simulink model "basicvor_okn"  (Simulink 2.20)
settings: Solver=ode45  StartTime=0  StopTime=10  MaxStep=.1  RelTol=1e-3  AbsTol=1e-3
undefined symbols (not defined in the file or in its folder): sfuny

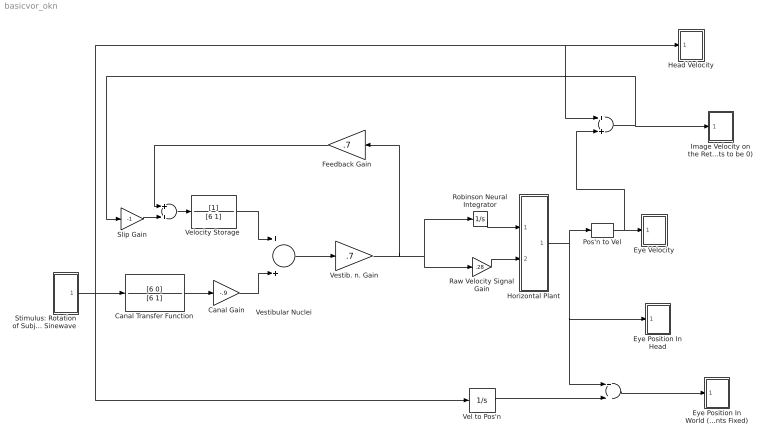
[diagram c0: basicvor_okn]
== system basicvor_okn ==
  " " : Sum  Inputs=++
  "  " : Sum  Inputs=++
  "   " : Sum  Inputs=++
  Canal Transfer Function : TransferFcn  Numerator=[6 0]  Denominator=[6 1]
  Canal Gain : Gain  Gain=-.9
  Eye Position In Head : Subsystem  LoadFcn=sfuny([],[],[],'LoadBlock')  StartFcn=sfuny([],[],[],'Start')  StopFcn=sfuny([],[],[],'Stop')  mask(Graph scope.){}
      mask help: Graph scope using MATLAB graph window. Enter plotting ranges and line type.
      mask init:
      | color = @4; ax = [0, @1, @2, @3]; dt = -1;
  Eye Position In World (Wants Fixed) : Subsystem  LoadFcn=sfuny([],[],[],'LoadBlock')  StartFcn=sfuny([],[],[],'Start')  StopFcn=sfuny([],[],[],'Stop')  mask(Graph scope.){}
      mask help: Graph scope using MATLAB graph window. Enter plotting ranges and line type.
      mask init:
      | color = @4; ax = [0, @1, @2, @3]; dt = -1;
  Eye Velocity : Subsystem  LoadFcn=sfuny([],[],[],'LoadBlock')  StartFcn=sfuny([],[],[],'Start')  StopFcn=sfuny([],[],[],'Stop')  mask(Graph scope.){}
      mask help: Graph scope using MATLAB graph window. Enter plotting ranges and line type.
      mask init:
      | color = @4; ax = [0, @1, @2, @3]; dt = -1;
  Feedback Gain : Gain  Orientation=left  Gain=.7
  Head Velocity : Subsystem  LoadFcn=sfuny([],[],[],'LoadBlock')  StartFcn=sfuny([],[],[],'Start')  StopFcn=sfuny([],[],[],'Stop')  mask(Graph scope.){}
      mask help: Graph scope using MATLAB graph window. Enter plotting ranges and line type.
      mask init:
      | color = @4; ax = [0, @1, @2, @3]; dt = -1;
  Horizontal Plant : Subsystem
  Image Velocity on the Retina (wants to be 0) : Subsystem  LoadFcn=sfuny([],[],[],'LoadBlock')  StartFcn=sfuny([],[],[],'Start')  StopFcn=sfuny([],[],[],'Stop')  mask(Graph scope.){}
      mask help: Graph scope using MATLAB graph window. Enter plotting ranges and line type.
      mask init:
      | color = @4; ax = [0, @1, @2, @3]; dt = -1;
  Pos'n to Vel : Derivative
  Raw Velocity Signal Gain : Gain  Gain=.28
  Robinson Neural Integrator : Integrator  ExternalReset=none  InitialConditionSource=internal  InitialCondition=0  LimitOutput=off  UpperSaturationLimit=inf  LowerSaturationLimit=-inf  ShowSaturationPort=off  ShowStatePort=off  AbsoluteTolerance=auto
  Slip Gain : Gain  Gain=-1
  Stimulus: Rotation of Subject Either Velocity Step or Sinewave : Subsystem
  Vel to Pos'n : Integrator  ExternalReset=none  InitialConditionSource=internal  InitialCondition=0  LimitOutput=off  UpperSaturationLimit=inf  LowerSaturationLimit=-inf  ShowSaturationPort=off  ShowStatePort=off  AbsoluteTolerance=auto
  "Velocity Storage " : TransferFcn  Numerator=[1]  Denominator=[6 1]
  Vestib. n. Gain : Gain  Gain=.7
  Vestibular Nuclei : Sum  Inputs=++
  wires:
  Canal Gain/1 -> Vestibular Nuclei/2
  Canal Transfer Function/1 -> Canal Gain/1
  "Velocity Storage "/1 -> Vestibular Nuclei/1
  Vestibular Nuclei/1 -> Vestib. n. Gain/1
  Vestib. n. Gain/1 -> Feedback Gain/1, Raw Velocity Signal Gain/1, Robinson Neural Integrator/1
  Raw Velocity Signal Gain/1 -> Horizontal Plant/2(in_2)
  Robinson Neural Integrator/1 -> Horizontal Plant/1(in_1)
  Horizontal Plant/1(out_1) -> Pos'n to Vel/1, Eye Position In Head/1(x), "   "/1
  Pos'n to Vel/1 -> Eye Velocity/1(x), "  "/2
  Stimulus: Rotation of Subject Either Velocity Step or Sinewave/1(out_1) -> Vel to Pos'n/1, Head Velocity/1(x), "  "/1, Canal Transfer Function/1
  "   "/1 -> Eye Position In World (Wants Fixed)/1(x)
  Vel to Pos'n/1 -> "   "/2
  " "/1 -> "Velocity Storage "/1
  Feedback Gain/1 -> " "/1
  "  "/1 -> Image Velocity on the Retina (wants to be 0)/1(x), Slip Gain/1
  Slip Gain/1 -> " "/2

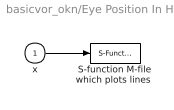
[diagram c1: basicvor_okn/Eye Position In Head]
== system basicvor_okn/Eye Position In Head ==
  x : Inport  Port=1  PortWidth=-1  SampleTime=-1
  "S-function M-file which plots lines " : S-Function  FunctionName=sfuny  Parameters=ax, color,dt  PortCounts=[]  SFunctionModules=''
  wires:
  x/1 -> "S-function M-file which plots lines "/1

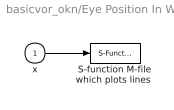
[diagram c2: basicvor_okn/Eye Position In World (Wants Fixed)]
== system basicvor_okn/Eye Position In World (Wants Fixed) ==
  x : Inport  Port=1  PortWidth=-1  SampleTime=-1
  "S-function M-file which plots lines " : S-Function  FunctionName=sfuny  Parameters=ax, color,dt  PortCounts=[]  SFunctionModules=''
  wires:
  x/1 -> "S-function M-file which plots lines "/1

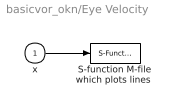
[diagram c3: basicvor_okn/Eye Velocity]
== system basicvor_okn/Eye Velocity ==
  x : Inport  Port=1  PortWidth=-1  SampleTime=-1
  "S-function M-file which plots lines " : S-Function  FunctionName=sfuny  Parameters=ax, color,dt  PortCounts=[]  SFunctionModules=''
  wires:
  x/1 -> "S-function M-file which plots lines "/1

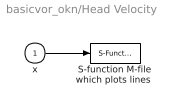
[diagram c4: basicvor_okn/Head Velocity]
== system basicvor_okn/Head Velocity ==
  x : Inport  Port=1  PortWidth=-1  SampleTime=-1
  "S-function M-file which plots lines " : S-Function  FunctionName=sfuny  Parameters=ax, color,dt  PortCounts=[]  SFunctionModules=''
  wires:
  x/1 -> "S-function M-file which plots lines "/1

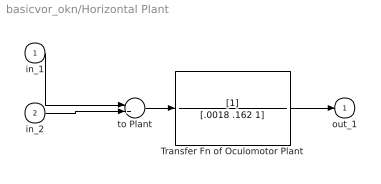
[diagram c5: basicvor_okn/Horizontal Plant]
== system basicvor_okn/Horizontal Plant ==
  in_1 : Inport  Port=1  PortWidth=-1  SampleTime=-1
  in_2 : Inport  Port=2  PortWidth=-1  SampleTime=-1
  Transfer Fn of Oculomotor Plant : TransferFcn  Numerator=[1]  Denominator=[.0018 .162 1]
  to Plant : Sum  Inputs=++
  out_1 : Outport  Port=1  InitialOutput=0
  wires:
  Transfer Fn of Oculomotor Plant/1 -> out_1/1
  in_2/1 -> to Plant/2
  in_1/1 -> to Plant/1
  to Plant/1 -> Transfer Fn of Oculomotor Plant/1

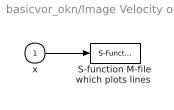
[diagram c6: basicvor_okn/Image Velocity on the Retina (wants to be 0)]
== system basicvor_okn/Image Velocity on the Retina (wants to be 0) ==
  x : Inport  Port=1  PortWidth=-1  SampleTime=-1
  "S-function M-file which plots lines " : S-Function  FunctionName=sfuny  Parameters=ax, color,dt  PortCounts=[]  SFunctionModules=''
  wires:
  x/1 -> "S-function M-file which plots lines "/1

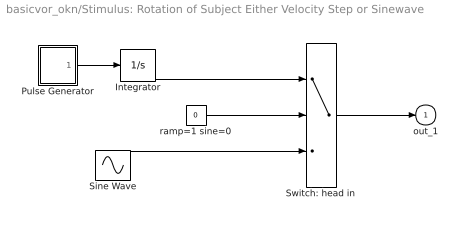
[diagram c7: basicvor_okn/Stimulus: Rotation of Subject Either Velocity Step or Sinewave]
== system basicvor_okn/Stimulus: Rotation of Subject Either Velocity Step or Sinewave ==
  Integrator : Integrator  ExternalReset=none  InitialConditionSource=internal  InitialCondition=0  LimitOutput=off  UpperSaturationLimit=inf  LowerSaturationLimit=-inf  ShowSaturationPort=off  ShowStatePort=off  AbsoluteTolerance=auto
  Pulse Generator : Subsystem  mask(Pulse Generator){}
      mask help: Pulse Generator.
      mask init:
      | Ts=@1; du=@2; ht=@3; stt=@4; ini=ones(length(ht),1); st1=rem(stt,Ts); st2=rem(stt+du,Ts);if(Ts<=1.2*du),ini=zeros(length(ht),1);end;
  Sine Wave : Sin  Amplitude=40  Frequency=.01*pi*2  Phase=0  SampleTime=-1
  Switch: head in : Switch  Threshold=.5
  ramp=1 sine=0 : Constant  Value=0
  out_1 : Outport  Port=1  InitialOutput=0
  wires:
  Switch: head in/1 -> out_1/1
  Integrator/1 -> Switch: head in/1
  Sine Wave/1 -> Switch: head in/3
  ramp=1 sine=0/1 -> Switch: head in/2
  Pulse Generator/1(out_1) -> Integrator/1

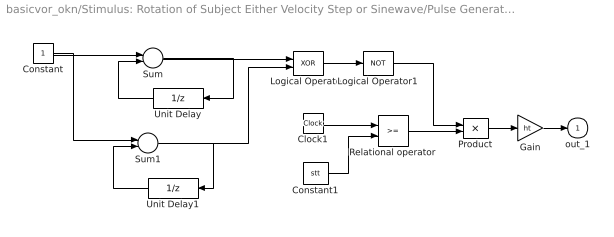
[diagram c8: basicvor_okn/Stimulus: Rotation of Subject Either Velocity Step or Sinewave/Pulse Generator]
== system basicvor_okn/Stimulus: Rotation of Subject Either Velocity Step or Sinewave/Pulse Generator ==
  Clock1 : Clock
  Constant : Constant  Value=1
  Constant1 : Constant  Value=stt
  Gain : Gain  Gain=ht
  Logical Operator : Logic  Operator=XOR  Inputs=2
  Logical Operator1 : Logic  Operator=NOT  Inputs=1
  Product : Product  Inputs=2
  Relational operator : RelationalOperator  Operator=>=
  Sum : Sum  Inputs=+-
  Sum1 : Sum  Inputs=+-
  Unit Delay : UnitDelay  Orientation=left  X0=0  SampleTime=[Ts,st1]
  Unit Delay1 : UnitDelay  Orientation=left  X0=ini  SampleTime=[Ts,st2]
  out_1 : Outport  Port=1  InitialOutput=0
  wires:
  Sum1/1 -> Logical Operator/2, Unit Delay1/1
  Sum/1 -> Logical Operator/1, Unit Delay/1
  Constant/1 -> Sum1/1, Sum/1
  Unit Delay1/1 -> Sum1/2
  Unit Delay/1 -> Sum/2
  Clock1/1 -> Relational operator/1
  Relational operator/1 -> Product/2
  Product/1 -> Gain/1
  Gain/1 -> out_1/1
  Constant1/1 -> Relational operator/2
  Logical Operator/1 -> Logical Operator1/1
  Logical Operator1/1 -> Product/1
